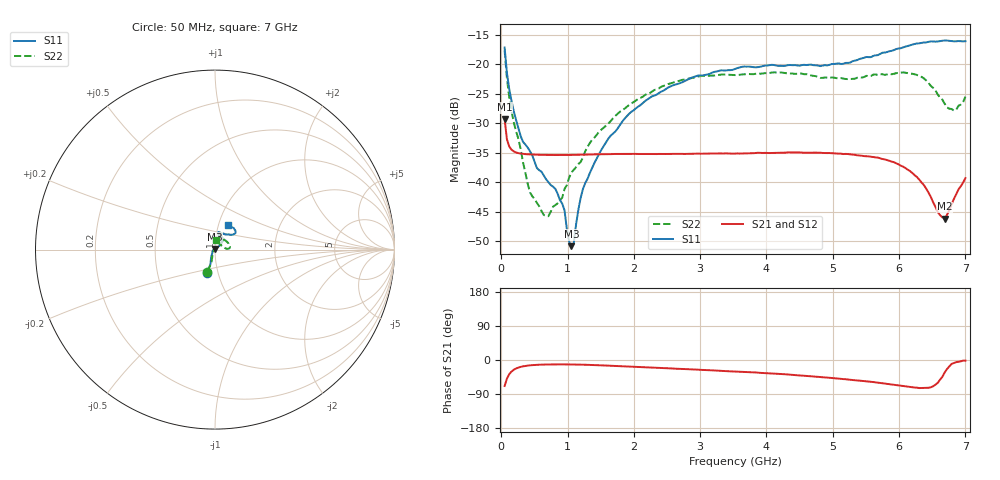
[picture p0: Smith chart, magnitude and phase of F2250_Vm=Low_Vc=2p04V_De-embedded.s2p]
! Integrated Device Technology
! Corporate Headquarters
! 6024 Silver Creek Valley Road
! San Jose, CA 95138  USA
! Phone:  1-408-284-8200
! Toll Free:  1-800-223-1366
! Webpage:  http://www.idt.com/
! Timing and RF Division
! 515 Groton Road, Suite 102
! Westford, MA 01886-6024
! Device:  F2250
! Description: Voltage Variable RF Attenuator
! Frequency:  50.0 -  6000.00 MHz
! Package:  3x3 mm Thin QFN Plastic Package: 16 pin
! Ports:  2 RF, 3 DC
!  Pin  1  = GND
!  Pin  2  = NC
!  Pin  3  = RF1  = Port 1
!  Pin  4  = NC
!  Pin  5  = GND
!  Pin  6  = GND
!  Pin  7  = GND
!  Pin  8  = GND
!  Pin  9  = NC
!  Pin 10  = RF2  = Port 2
!  Pin 11  = NC
!  Pin 12  = GND
!  Pin 13  = GND
!  Pin 14  = VCNTRL
!  Pin 15  = VDD
!  Pin 16  = VMODE
! Vcntrl:  2.040 Volts
! Vmode:  +0.000 Volts
! Vdd:  +3.30  Volts
! Current:  1.184 mA
! Data:  The device was measured on a the F2250 evaluation board which has
!  individual transmission lines to the RF pins.  Data was collected
!  using a calibrated network analyzer.  The evaluation board was
!  de-embedded using a TRL calibration technique.
!  The reference plane is the edge of the package pin.
! Misc:  SN 10
!  Action Tracker AT0258
! Date Measured:  2014-11-26
! Date:  2015-10-15  MJV
! Note:
!  Integrated Device Technology supplies this data as a sample of measured
!  data at the package pin for this product.  Your particular data for this
!  product may vary.
!  Data was taken at 25 degrees C.
!  Integrated Device Technology reserves the right to change this data at anytime.
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# GHz S dB R 50
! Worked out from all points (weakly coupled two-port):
!   201 points, 50 MHz to 7 GHz, reference 50 ohm
!   highest |S21| = -29.30 dB at 50 MHz (marker M1); lowest = -46.2 dB at 6.687 GHz (marker M2)
!   lowest |S11| = -50.8 dB at 1.058 GHz (marker M3), VSWR 1.01, Z = 49.8 + j0.241 ohm
!   |S11| at or under -10 dB: start of sweep to end of sweep
!   |S22| runs from -45.7 to -17.7 dB; largest |S21 - S12| = 6.7e-05
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0.05  -17.18 -108.6  -29.30 -68.6  -29.30 -68.6  -17.69 -109.0
0.08475  -21.44 -107.4  -32.71 -49.3  -32.71 -49.2  -22.34 -105.2
0.189  -28.00 -119.6  -34.77 -25.6  -34.77 -25.7  -29.87 -114.9
0.29325  -32.20 -127.7  -35.13 -18.1  -35.13 -18.1  -34.44 -119.0
0.43225  -34.72 -144.5  -35.28 -14.1  -35.27 -14.1  -41.69 -150.6
0.71025  -39.97 -168.5  -35.36 -11.8  -35.36 -11.8  -45.73 132.3
0.91875  -43.60 158.1  -35.37 -11.6  -35.37 -11.6  -42.60 92.8
0.9535  -44.72 170.3  -35.37 -11.6  -35.37 -11.7  -41.13 95.7
1.023  -50.02 143.9  -35.36 -11.7  -35.37 -11.8  -39.21 78.0
1.05775  -50.80 123.1  -35.36 -11.8  -35.36 -11.8  -38.30 74.3
1.0925  -50.34 89.0  -35.35 -11.9  -35.35 -11.9  -37.90 69.9
1.162  -44.65 56.3  -35.33 -12.1  -35.33 -12.1  -36.90 60.5
1.2315  -41.12 44.3  -35.30 -12.4  -35.30 -12.4  -35.78 53.5
1.6485  -32.11 41.9  -35.22 -15.0  -35.22 -15.0  -29.65 48.8
2.37825  -24.87 47.3  -35.19 -20.8  -35.19 -20.8  -24.09 48.7
3.525  -20.80 72.5  -35.13 -30.2  -35.13 -30.3  -21.85 70.6
4.7065  -20.17 72.3  -34.95 -43.4  -34.95 -43.4  -21.98 69.9
5.85325  -17.82 40.4  -36.35 -63.9  -36.35 -64.0  -21.67 18.7
6.33975  -16.40 41.0  -40.04 -73.9  -40.05 -73.9  -22.16 4.5
6.68725  -15.99 48.8  -46.17 -32.9  -46.13 -32.5  -26.69 24.7
6.861  -16.13 55.1  -42.03 -5.7  -41.99 -5.7  -27.73 58.5
7  -16.12 63.2  -39.28 -1.6  -39.24 -1.7  -25.49 86.4
